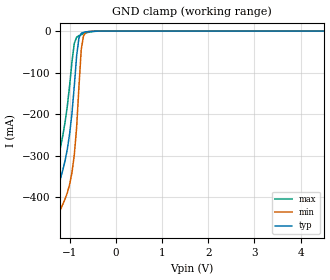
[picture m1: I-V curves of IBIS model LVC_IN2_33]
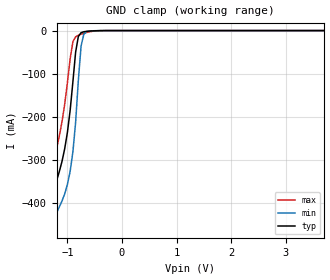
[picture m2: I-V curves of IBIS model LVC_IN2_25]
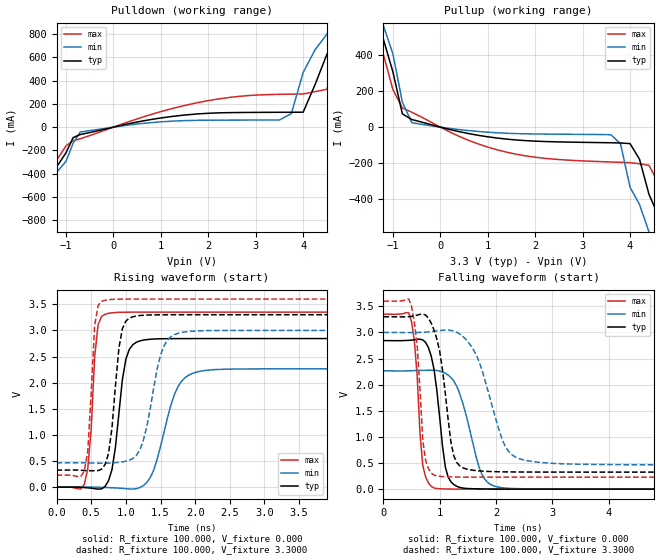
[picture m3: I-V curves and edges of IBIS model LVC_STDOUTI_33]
| Philips Semiconductors Inc.
| Logic Products Group
| IBIS model of 74LVC04A
|  HEX INVERTER
|[Packages]:
|[Package1]: SO 14-pin (D) Package ;
|[Package2]: SSOP 14-Pin Packages ;
|[Package3]: TSSOP 14-pin (PW) Package ;
[IBIS Ver]   3.2
[File Name]   lvc04a.ibs
[File Rev]   1.2
[Date]   26-Nov-2002
[Source]   File created from simulations by LPG
   Philips Semiconductors Nijmegen
[Notes]   V1.2   Ibis model.
| Remark:
| The Power Clamp curves have been omitted since there is no power clamp diode.
| Revision History
| Version Date   Author/ Description
|   Editor
| 1.0   1999   Initial Version
| 1.1   November 2001 RM   Revised for Ibis 3.2:
|   Added Model Spec and Model Selector
| 1.2   November 2002 RM   Revised: Power Clamp curves omitted, constant
|   end points for Ground Clamp and V/t curves.
[Disclaimer]
   (C) Copyright 2002 Philips Semiconductors
   All rights reserved
   Philips Semiconductors warrants and represents that the IBIS model
   identified herein is owned by Philips Semiconductors (PHILIPS). The
   model provided is not warranted as fully representing all of the
   operating characteristics and specifications of the semiconductor
   products to which the model relates.  Moreover, unless there is a
   signed, written agreement to the contrary, this IBIS model is
   furnished on an "as is" basis without support or warranty of any
   kind, either expressed or implied, regarding the use thereof, and
   PHILIPS specifically disclaims all implied warranties of
   merchantability and fitness of the model for any purpose.
   PHILIPS does not assume any liability arising out of the application
   or use of this IBIS model including infringement of patents and
   copyrights, nor does PHILIPS convey any license under its patents and
   copyrights or the rights of others.
   PHILIPS provides IBIS models as a service to our customers. You and
   your company shall not distribute, convey, sell, or give these models
   to anyone else without receiving prior written permission from
   PHILIPS.
   PHILIPS reserves the right to make changes without notice to these
   IBIS models to improve reliability, function, or design.
   Please be aware that your receipt and subsequent use of the IBIS
   information provided shall serve as acceptance of the terms and
   conditions of this agreement.  If you do not accept these terms,
   you should return or destroy the IBIS models and any other
   accompanying information immediately.
| to specify a consistent format that can be parsed by software, allowing
| simulation vendors to derive models compatible with their own products.
| One goal of this template is to represent the current state of IBIS data,
| while allowing a growth path to more complex models / methods (when deemed
| appropriate).  This would be accomplished by a revision of the base
| template, and possibly the addition of new keywords or categories.
| Another goal of this template is to ensure that it is simple enough for
| semiconductor vendors and customers to use and modify, while ensuring that
| it is rigid enough for simulation vendors to write reliable parsers.
| Finally, this template is meant to contain a complete description of the I/O
| elements on an entire component.  Consequently, several models will need to
| be defined in each file, as well as a table that equates the appropriate
| buffer to the correct pin and signal name.
| Version 3.2 of this electronic template was finalized by an industry-wide
| group of experts representing various companies and interests.  Regular
| "EIA IBIS Open Forum" meetings were held to accomplish this task.
| Commitment to Backward Compatibility.  Version 1.0 is the first valid IBIS
| ASCII file format.  It represents the minimum amount of I/O buffer
| information required to create an accurate IBIS model of common CMOS and
| bipolar I/O structures.  Future revisions of the ASCII file will add items
| considered to be "enhancements" to Version 1.0 to allow accurate modeling
| of new, or other I/O buffer structures.  Consequently, all future revisions
| will be considered supersets of Version 1.0, allowing backward
| compatibility.  In addition, as modeling platforms develop support for
| revisions of the IBIS ASCII template, all previous revisions of the template
| must also be supported.
| Version 1.1 update.  The file "ver1_1.ibs" is conceptually the same as the
| 1.0 version of the IBIS ASCII format (ver1_0.ibs).  However, various
| comments have been added for further clarification.
| Version 2.0 update.  The file "ver2_0.ibs" maintains backward compatibility
| with Versions 1.0 and 1.1.  All new keywords and elements added in Version
| 2.0 are optional.  A complete list of changes to the specification is in the
| IBIS Version 2.0 Release Notes document ("ver2_0.rn").
| Version 2.1 update.  The file "ver2_1.ibs" contains clarification text
| changes, corrections, and two additional waveform parameters beyond
| Version 2.0.
| Version 3.0 update.  The file "ver3_0.ibs" adds a number of new keywords
| and functionality.  A complete list of functions can be found on eda.org
| under /pub/ibis/birds/birddir.txt showing the approved Buffer Issue
| Resolution Documents (BIRDs) that have been approved for Version 3.0.
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[Component]   74LVC04A_1
[Manufacturer]   Philips Semiconductors Inc.
[Package]
|   typ   min   max
R_pkg   4.54E-02   4.18E-02   5.01E-02
L_pkg   2.31E-09   1.63E-09   3.26E-09
C_pkg   0.565E-12  0.437E-12  0.736E-12
[Pin] signal_name   model_name   R_pin   L_pin   C_pin
   1   1A   lvc_in2 4.18E-02 3.26E-09 0.675E-12
   2   1Y#   lvc_stdouti 5.01E-02 2.30E-09 0.574E-12
   3   2A   lvc_in2 4.52E-02 1.71E-09 0.467E-12
   4   2Y#   lvc_stdouti 4.38E-02 1.63E-09 0.437E-12
   5   3A   lvc_in2 4.52E-02 1.71E-09 0.465E-12
   6   3Y#   lvc_stdouti 5.01E-02 2.30E-09 0.573E-12
   7   GND   GND 4.18E-02 3.26E-09 0.736E-12
   8   4Y#   lvc_stdouti 4.18E-02 3.26E-09 0.736E-12
   9   4A   lvc_in2 5.01E-02 2.30E-09 0.573E-12
   10   5Y#   lvc_stdouti 4.52E-02 1.71E-09 0.465E-12
   11   5A   lvc_in2 4.38E-02 1.63E-09 0.437E-12
   12   6Y#   lvc_stdouti 4.52E-02 1.71E-09 0.467E-12
   13   6A   lvc_in2 5.01E-02 2.30E-09 0.574E-12
   14   VCC   POWER 4.18E-02 3.26E-09 0.736E-12
|   Info for  SSOP 14-Pin Packages
[Component]   74LVC04A_2
[Manufacturer]   Philips Semiconductors Inc.
[Package]
|   typ   min   max
R_pkg   18.10E-03   15.70E-03   19.10E-03
L_pkg   2.12E-09   1.76E-09   2.65E-09
C_pkg   0.59E-12   0.55E-12   0.64E-12
[Pin] signal_name   model_name   R_pin   L_pin   C_pin
   1   1A   lvc_in2 19.10E-03 2.65E-09 0.58E-12
   2   1Y#   lvc_stdouti 17.70E-03 2.07E-09 0.64E-12
   3   2A   lvc_in2 18.70E-03 1.82E-09 0.57E-12
   4   2Y#   lvc_stdouti 15.70E-03 1.76E-09 0.55E-12
   5   3A   lvc_in2 18.70E-03 1.82E-09 0.57E-12
   6   3Y#   lvc_stdouti 17.70E-03 2.07E-09 0.63E-12
   7   GND   GND 19.10E-03 2.65E-09 0.60E-12
   8   4Y#   lvc_stdouti 19.10E-03 2.65E-09 0.60E-12
   9   4A   lvc_in2 17.80E-03 2.07E-09 0.64E-12
   10   5Y#   lvc_stdouti 18.70E-03 1.82E-09 0.57E-12
   11   5A   lvc_in2 15.70E-03 1.76E-09 0.55E-12
   12   6Y#   lvc_stdouti 18.70E-03 1.82E-09 0.57E-12
   13   6A   lvc_in2 17.80E-03 2.07E-09 0.64E-12
   14   VCC   POWER 19.10E-03 2.65E-09 0.60E-12
|   Info for  TSSOP 14-pin (PW) Package
[Component]   74LVC04A_3
[Manufacturer]   Philips Semiconductors Inc.
[Package]
|   typ   min   max
R_pkg   3.44E-02   2.80E-02   4.33E-02
L_pkg   1.83E-09   1.36E-09   2.32E-09
C_pkg   0.380E-12  0.302E-12  0.442E-12
[Pin] signal_name   model_name   R_pin   L_pin   C_pin
   1   1A   lvc_in2 3.46E-02 2.32E-09 0.423E-12
   2   1Y#   lvc_stdouti 4.33E-02 2.04E-09 0.441E-12
   3   2A   lvc_in2 2.80E-02 1.36E-09 0.307E-12
   4   2Y#   lvc_stdouti 2.88E-02 1.38E-09 0.302E-12
   5   3A   lvc_in2 2.80E-02 1.36E-09 0.308E-12
   6   3Y#   lvc_stdouti 4.33E-02 2.04E-09 0.441E-12
   7   GND   GND 3.46E-02 2.32E-09 0.433E-12
   8   4Y#   lvc_stdouti 3.46E-02 2.32E-09 0.433E-12
   9   4A   lvc_in2 4.33E-02 2.04E-09 0.441E-12
   10   5Y#   lvc_stdouti 2.80E-02 1.36E-09 0.308E-12
   11   5A   lvc_in2 2.88E-02 1.38E-09 0.302E-12
   12   6Y#   lvc_stdouti 2.80E-02 1.36E-09 0.308E-12
   13   6A   lvc_in2 4.33E-02 2.04E-09 0.442E-12
   14   VCC   POWER 3.46E-02 2.31E-09 0.433E-12
[Model Selector]   lvc_in2
| Remark: If your software does not support the Model Selector
|   Please comment out the lines of the Model Selector, which
|   contain the name of the Model, except the one you want to use.
LVC_IN2_33   3.3V-Vcc input model
LVC_IN2_25   2.5V-Vcc input model
[Model Selector]   lvc_stdouti
| Remark: If your software does not support the Model Selector
|   Please comment out the lines of the Model Selector, which
|   contain the name of the Model, except the one you want to use.
LVC_STDOUTI_33   3.3V-Vcc inverting output model
LVC_STDOUTI_25   2.5V-Vcc inverting output model
| Models and submodels in the file (4): LVC_IN2_33 (Input), LVC_IN2_25 (Input), LVC_STDOUTI_33 (Output), LVC_STDOUTI_25 (Output)
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|   Model LVC_IN2_33
[Model]   LVC_IN2_33
Model_type   Input
Vinl =   0.8000V
Vinh =   2.0000V
C_comp   2.78pF   1.99pF   3.72pF
[Model Spec]
| Note: The input and output voltage ratings may be exceeded if the input and
|   output current ratings are observed (please refer to the data sheet)
|   Subparameter   typ   min   max
| Thresholds
Vinh   2.0   NA   NA
Vinl   0.8   NA   NA
| Overshoot
S_overshoot_high   6.5   6.5   6.5   | Static overshoot
S_overshoot_low   -0.5   -0.5   -0.5
D_overshoot_high   7.2   7.2   7.2   | Dynamic overshoot
D_overshoot_low   -0.95   -0.9   -1.0
D_overshoot_time   3n   3n   3n
|Ambient temperature:   25.0000   85.0000   -40.0000
[Temperature Range]   40.0000   100.0000   -25.0000
[Voltage Range]   3.3000V   3.0000V   3.6000V
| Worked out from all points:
|   GND clamp passes 1 mA (typ) near -0.57 V on its own axis
|Process Range   nominal   slow   fast
[GND_clamp]
| voltage   I(typ)   I(min)   I(max)
-5.5V     -4.567A    -4.624A    -4.51A
-1.45V    -555.2mA   -621.5mA   -488.4mA
-1.35V    -461.8mA   -528.7mA   -394.3mA
-1.3V     -417.5mA   -485mA     -349.4mA
-1.1V     -312.4mA   -404.8mA   -219.8mA
-950mV    -197.3mA   -340.4mA   -73.13mA
-900mV    -132mA     -298.5mA   -29.44mA
-850mV    -59.79mA   -233mA     -14.94mA
-800mV    -16.87mA   -135mA     -10.93mA
-750mV    -5.479mA   -44.49mA   -8.487mA
-700mV    -2.88mA    -11.01mA   -6.407mA
5.5V      1.567nA    9.324nA    202.5pA
|   Model LVC_IN2_25
[Model]   LVC_IN2_25
Model_type   Input
Vinl =   0.7000V
Vinh =   1.7000V
C_comp   2.84pF   2.10pF   3.71pF
[Model Spec]
| Note: The input and output voltage ratings may be exceeded if the input and
|   output current ratings are observed (please refer to the data sheet)
|   Subparameter   typ   min   max
| Thresholds
Vinh   1.7   NA   NA
Vinl   0.7   NA   NA
| Overshoot
S_overshoot_high   6.5   6.5   6.5   | Static overshoot
S_overshoot_low   -0.5   -0.5   -0.5
D_overshoot_high   7.2   7.2   7.2   | Dynamic overshoot
D_overshoot_low   -0.95   -0.9   -1.0
D_overshoot_time   3n   3n   3n
|Ambient temperature:   25.0000   85.0000   -40.0000
[Temperature Range]   35.0000   95.0000   -30.0000
[Voltage Range]   2.5000V   2.3000V   2.7000V
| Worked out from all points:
|   GND clamp passes 1 mA (typ) near -0.57 V on its own axis
|Process Range   nominal   slow   fast
[GND_clamp]
| voltage   I(typ)   I(min)   I(max)
-5.5V     -4.558A    -4.615A    -4.502A
-1.45V    -549mA     -615mA     -482.5mA
-1.35V    -455.6mA   -522.2mA   -388.4mA
-1.3V     -411.3mA   -478.6mA   -343.5mA
-1.1V     -304mA     -396mA     -212mA
-950mV    -185.1mA   -326.6mA   -65.02mA
-900mV    -119.1mA   -281.8mA   -26.08mA
-850mV    -50.24mA   -213.2mA   -14.46mA
-800mV    -13.81mA   -116mA     -10.88mA
-750mV    -4.865mA   -35.92mA   -8.446mA
-700mV    -2.732mA   -8.828mA   -6.333mA
5.5V      922.9pA    6.4nA      86.94pA
|   Model LVC_STDOUTI_33
[Model]   LVC_STDOUTI_33
Model_type   Output
Polarity   Inverting
Vmeas =  1.5000V
Cref  = 50.0000pF
Rref  =  0.5000k
Vref  =  0.000V
C_comp   2.75pF   1.80pF   3.60pF
[Model Spec]
| Note: The input and output voltage ratings may be exceeded if the input and
|   output current ratings are observed (please refer to the data sheet)
|   Subparameter   typ   min   max
| Timing Thresholds
Vmeas   1.5   1.5   1.5
|Ambient temperature:   25.0000   85.0000   -40.0000
[Temperature Range]   40.0000   100.0000   -25.0000
[Voltage Range]   3.3000V   3.0000V   3.6000V
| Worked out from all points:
|   slope of the pulldown table from 0 to 0.495 V, typ, clamps not added: 11.4 ohm
|   slope of the pullup table from 0 to 0.495 V, typ, clamps not added: 16.3 ohm
|   rising waveform, R_fixture 100.000, V_fixture 0.000: 20-80 % time 151ps typ, 281ps min, 93.8ps max; typ from 0 V to 2.84 V
|   rising waveform, R_fixture 100.000, V_fixture 3.3000: 20-80 % time 127ps typ, 227ps min, 83.5ps max; typ from 0.327 V to 3.3 V
|   falling waveform, R_fixture 100.000, V_fixture 0.000: 20-80 % time 180ps typ, 331ps min, 120ps max; typ from 2.84 V to 0 V
|   falling waveform, R_fixture 100.000, V_fixture 3.3000: 20-80 % time 212ps typ, 424ps min, 123ps max; typ from 3.3 V to 0.327 V
|Process Range   nominal   slow   fast
[Pulldown]
| voltage   I(typ)   I(min)   I(max)
-5.5V     -4.54A     -4.575A    -4.499A
-1.9V     -965.6mA   -1.008A    -916.3mA
-1.75V    -819.9mA   -862.8mA   -770.1mA
-1.3V     -396.9mA   -441.3mA   -346.7mA
-700mV    -63.6mA    -42.24mA   -99.98mA
3.5V      127.9mA    61.26mA    282.4mA
3.75V     128.1mA    116.3mA    283.9mA
4V        128.6mA    470mA      285mA
4.5V      626.2mA    799.3mA    325.7mA
4.75V     782.6mA    1.022A     641.1mA
5.25V     1.25A      1.523A     1.047A
11V       6.838A     7.162A     6.537A
[Pullup]
| voltage   I(typ)   I(min)   I(max)
-8V       7.121A     7.153A     7.096A
-1.6V     743.1mA    797.9mA    680.6mA
-1.2V     489.6mA    565.9mA    404.2mA
-800mV    73.9mA     139.3mA    106.7mA
-600mV    42.4mA     24.62mA    82.79mA
1.4V      -66.79mA   -34.12mA   -139.7mA
3.6V      -87.04mA   -42.47mA   -194.3mA
3.8V      -88.38mA   -93.57mA   -196mA
4V        -91.76mA   -334.9mA   -198.2mA
4.4V      -374.8mA   -584.4mA   -213.2mA
5V        -890.3mA   -1.178A    -648.8mA
9.1V      -4.852A    -5.18A     -4.53A
[Ramp]
| variable   typ   min   max
dV/dt_r   1.706V/150.834ps   1.359V/281.363ps   2.010V/93.759ps
dV/dt_f   1.784V/211.753ps   1.521V/423.765ps   2.022V/122.938ps
R_load = 100.000
[Rising Waveform]
R_fixture   = 100.000
V_fixture   = 0.000
V_fixture_min = 0.000
V_fixture_max = 0.000
| time   V(typ)   V(min)   V(max)
0s        113.6pV    3.037nV    227.9pV
400ps     -7.454mV   1.677mV    49.33mV
500ps     -19.7mV    649uV      1.109V
600ps     -38.48mV   -2.249mV   3.112V
750ps     124.7mV    -9.005mV   3.327V
1ns       2.447V     -29.32mV   3.348V
1.25ns    2.814V     27.92mV    3.35V
1.75ns    2.843V     1.918V     3.35V
2.05ns    2.844V     2.212V     3.35V
9.75ns    2.844V     2.264V     3.35V
[Rising Waveform]
R_fixture   = 100.000
V_fixture   = 3.3000
V_fixture_min = 3.0000
V_fixture_max = 3.6000
| time   V(typ)   V(min)   V(max)
0s        326.6mV    465.6mV    230.2mV
400ps     318.4mV    465.8mV    306.3mV
450ps     315.2mV    464.6mV    678.1mV
550ps     314.7mV    461.4mV    3.092V
700ps     432.1mV    459.5mV    3.578V
950ps     3.032V     483.8mV    3.599V
1.1ns     3.261V     548mV      3.6V
1.55ns    3.299V     2.704V     3.6V
1.8ns     3.3V       2.959V     3.6V
9.75ns    3.3V       3V         3.6V
[Falling Waveform]
R_fixture   = 100.000
V_fixture   = 0.000
V_fixture_min = 0.000
V_fixture_max = 0.000
| time   V(typ)   V(min)   V(max)
0s        2.844V     2.264V     3.35V
500ps     2.852V     2.268V     3.205V
600ps     2.869V     2.272V     2.162V
700ps     2.857V     2.275V     444.8mV
900ps     2.286V     2.276V     22.51mV
1.1ns     422.5mV    2.218V     4.059mV
1.35ns    35.25mV    1.843V     820.9uV
1.75ns    4.652mV    281.2mV    70.19uV
2.05ns    1.645mV    37.4mV     11.4uV
9.75ns    113.7pV    35.97nV    227.9pV
[Falling Waveform]
R_fixture   = 100.000
V_fixture   = 3.3000
V_fixture_min = 3.0000
V_fixture_max = 3.6000
| time   V(typ)   V(min)   V(max)
0s        3.3V       3V         3.6V
500ps     3.307V     2.998V     3.497V
600ps     3.332V     3V         2.745V
700ps     3.352V     3.004V     927.1mV
900ps     3.042V     3.023V     268mV
1.25ns    638.2mV    3.026V     233mV
1.45ns    392.8mV    2.883V     231mV
2.15ns    331.3mV    850.1mV    230.2mV
2.45ns    328.3mV    571.2mV    230.2mV
9.75ns    326.6mV    465.6mV    230.2mV
